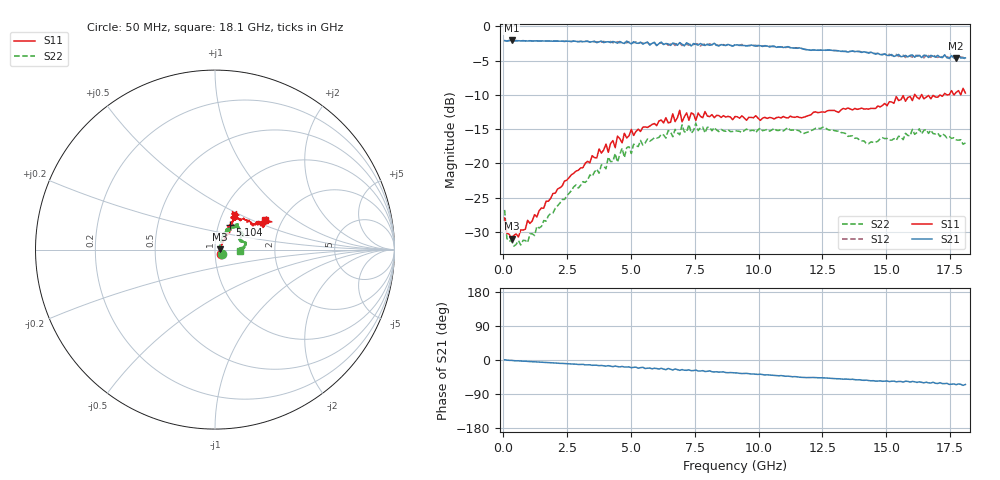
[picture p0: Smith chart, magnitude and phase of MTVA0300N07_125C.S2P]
! Network Analyzer HP8720D.06.14 Serial No. US36140669
! 27 Jun 2005  12:28:32
! Frequency  S11  S21  S12  S22
# HZ  S  DB R 50
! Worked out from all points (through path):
!   201 points, 50 MHz to 18.1 GHz, reference 50 ohm
!   highest |S21| = -2.07 dB at 320.8 MHz (marker M1); lowest = -4.7 dB at 17.74 GHz (marker M2)
!   group delay of S21, straight-line fit = 10.1 ps
!   lowest |S11| = -31.0 dB at 320.8 MHz (marker M3), VSWR 1.06, Z = 52.9 + j0.0619 ohm
!   |S11| at or under -10 dB: start of sweep to 16.11 GHz; 16.13 GHz to 16.38 GHz (250.5 MHz wide, 1.54 % of centre); 16.39 GHz to 17.24 GHz (853.9 MHz wide, 5.08 % of centre)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
!   |S22| runs from -32.1 to -14.2 dB; largest |S21 - S12| = 0.041
!   S11 on the Smith chart (normalised r, x): 50 MHz: 1.07, -0.05; 5.104 GHz: 1.13, +0.32; 18.1 GHz: 1.64, +0.61
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5e7  -27.98 -34.5  -2.09 0.5  -2.08 0.5  -26.81 -34.9
1.4025e8  -30.23 -18.1  -2.15 -0.3  -2.14 -0.3  -31.00 -20.2
3.2075e8  -30.99 1.2  -2.07 -0.9  -2.10 -0.9  -31.27 -3.3
9.525e8  -28.33 26.4  -2.14 -3.8  -2.10 -3.7  -31.59 25.3
3.1185e9  -20.63 51.4  -2.24 -11.5  -2.26 -11.9  -22.68 58.5
4.021e9  -17.19 55.0  -2.29 -16.2  -2.29 -15.1  -20.80 57.1
4.11125e9  -18.39 55.5  -2.25 -14.9  -2.36 -16.2  -19.08 57.5
4.47225e9  -16.04 51.8  -2.47 -17.3  -2.24 -16.6  -19.86 62.3
4.65275e9  -17.02 52.3  -2.40 -17.0  -2.30 -18.6  -17.79 61.7
4.743e9  -15.61 55.5  -2.50 -18.5  -2.38 -17.5  -19.18 58.0
5.104e9  -15.94 58.8  -2.25 -19.3  -2.39 -20.1  -17.21 54.4
6.09675e9  -13.83 57.4  -2.53 -23.8  -2.43 -23.5  -16.22 52.7
6.909e9  -12.27 60.5  -2.38 -27.3  -2.44 -25.4  -15.84 48.3
6.99925e9  -13.94 60.4  -2.61 -25.3  -2.81 -27.3  -14.40 49.0
7.36025e9  -12.63 55.5  -2.88 -28.2  -2.51 -27.4  -15.61 51.5
7.54075e9  -13.73 58.2  -2.62 -26.4  -2.53 -29.5  -14.15 49.7
9.075e9  -13.18 60.3  -2.73 -34.0  -2.71 -34.1  -15.25 35.5
1.21435e10  -12.56 47.3  -3.46 -46.1  -3.42 -46.3  -15.09 34.1
1.512175e10  -11.01 30.9  -4.26 -56.9  -4.08 -56.6  -16.60 18.5
1.6295e10  -10.62 24.5  -4.26 -57.5  -4.28 -60.7  -14.96 12.2
1.7739e10  -9.65 27.1  -4.67 -65.1  -4.71 -64.9  -16.58 4.7
1.81e10  -9.73 30.4  -4.61 -64.7  -4.77 -65.4  -17.02 -2.3
